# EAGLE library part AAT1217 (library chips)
A Simple boost converter
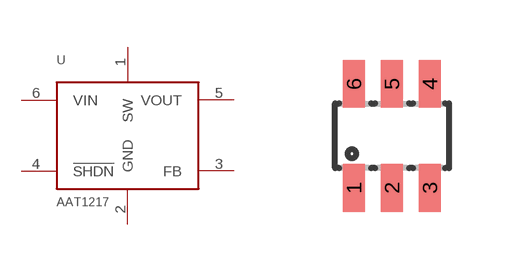
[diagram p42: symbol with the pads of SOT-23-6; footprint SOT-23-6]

Designator prefix U

## AAT12173.3V (DIGIKEY: 863-1496-1-ND)  [SOT-23-6]
1  SW
2  GND
3  FB
4  !SHDN
5  VOUT
6  VIN

## Footprint SOT-23-6 (pad centres in mm)
Small Outline Transistor
smd 0.55 x 1.2: 1 -0.95,-1.3; 2 0,-1.3; 3 0.95,-1.3; 4 0.95,1.3; 5 0,1.3; 6 -0.95,1.3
